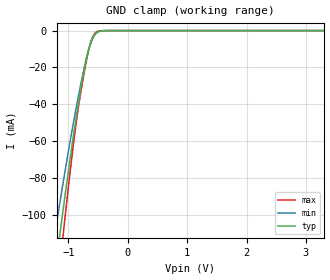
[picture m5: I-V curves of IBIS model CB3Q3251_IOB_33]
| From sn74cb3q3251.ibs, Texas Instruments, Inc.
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[Model]   CB3Q3251_IOB_33
Model_type  Terminator
| variable   typ   min   max
C_comp   16.75pF   13.18pF   20.32pF
| C_tri-state   16.75pF   13.18pF   20.32pF
[Temperature Range]   40   100   -40
| Ambient temperature   25   85   -40
[Voltage range]   3.3   3   3.6
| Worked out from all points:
|   GND clamp passes 1 mA (typ) near -0.51 V on its own axis
[GND Clamp]
| CB3Q3251_IOB_33
|   Voltage   I(typ)   I(min)   I(max)
-5.5V     -1.586A    -1.323A    -1.877A
-1.235V   -133.4mA   -112.1mA   -157.6mA
-1.2V     -124.5mA   -104.9mA   -146mA
-1.135V   -108.4mA   -91.66mA   -125.2mA
-1.1V     -99.88mA   -84.71mA   -114.4mA
-1.065V   -91.48mA   -77.85mA   -103.8mA
-900mV    -53.71mA   -47.25mA   -57.71mA
-790mV    -30.99mA   -28.82mA   -33.16mA
-650mV    -9.183mA   -9.516mA   -9.458mA
-540mV    -1.682mA   -1.708mA   -1.029mA
-310mV    -4.026uA   -7.614uA   -284.7nA
3.3V      519pA      1.779nA    106pA
